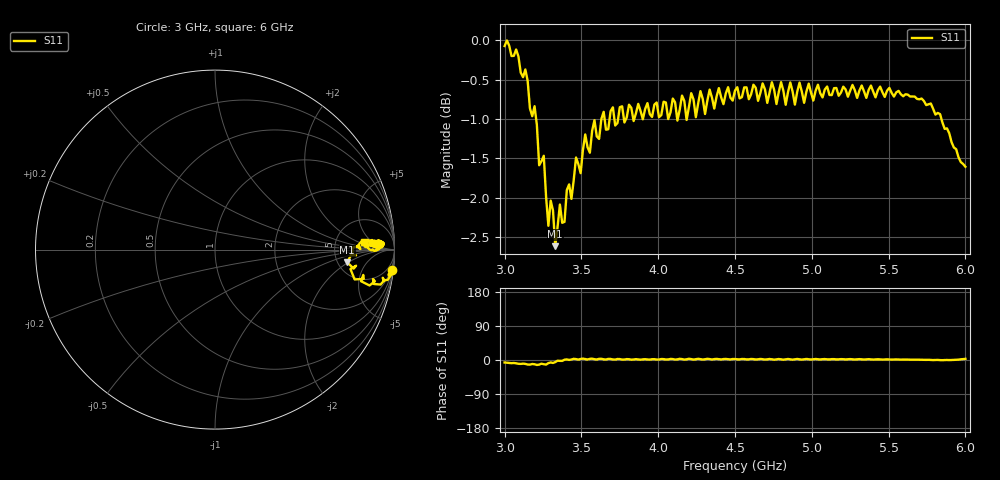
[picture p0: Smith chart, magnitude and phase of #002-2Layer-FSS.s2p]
!  05/08/2025  15:46:54
! Ref Plane: 0.000 mm
# MHZ S MA R  50
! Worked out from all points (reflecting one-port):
!   201 points, 3 GHz to 6 GHz, reference 50 ohm
!   lowest |S11| = -2.6 dB at 3.33 GHz (marker M1), VSWR 6.70, Z = 304 - j95.1 ohm
!   phase of S11 starts at -7 deg and turns +10 deg over the sweep
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3000  0.9919 -6.6
3135  0.9584 -10.3
3210  0.8838 -13.1
3225  0.8331 -12.2
3240  0.8381 -9.7
3255  0.8447 -11.2
3270  0.7953 -12.1
3285  0.7625 -8.2
3300  0.7911 -6.5
3330  0.7401 -5.5
3345  0.7615 -1.8
3375  0.7658 -2.3
3450  0.8153 3.1
3585  0.8899 2.1
3750  0.907 2.4
4125  0.8894 1.7
4155  0.9225 2.5
4185  0.8902 1.9
4215  0.9258 2.5
4245  0.8938 2.0
4275  0.9285 2.4
4305  0.898 2.2
4500  0.9293 2.6
4875  0.928 0.9
5250  0.9292 2.4
5625  0.9238 1.0
5895  0.873 -0.3
6000  0.8313 2.9
